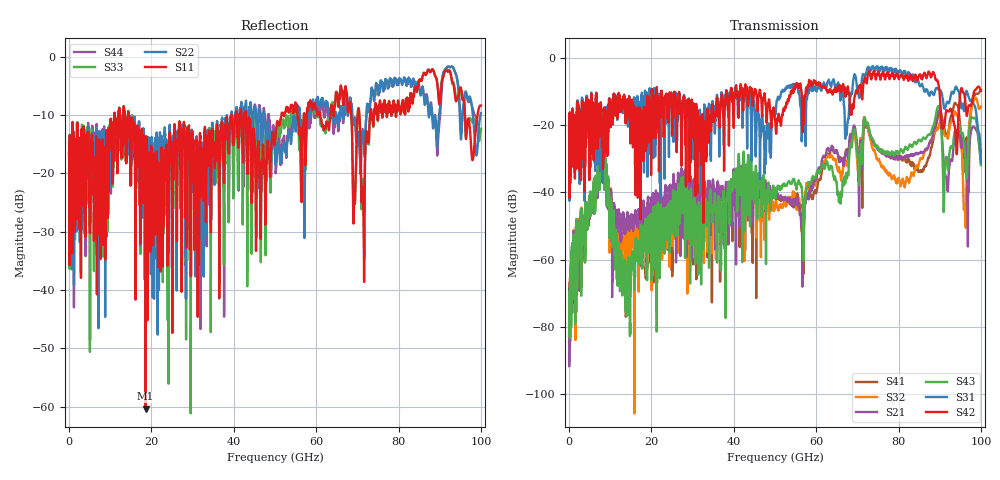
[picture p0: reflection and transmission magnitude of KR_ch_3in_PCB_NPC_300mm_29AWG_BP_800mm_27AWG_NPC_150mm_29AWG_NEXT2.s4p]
# GHz S RI R 45
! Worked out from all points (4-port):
!   4000 points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, 25 MHz to 100 GHz, reference 45 ohm
!   strongest paths, dB at 25 MHz, 25.02 GHz, 50.02 GHz, 75.03 GHz, 100 GHz:
!     S42: -21.2, -20.7, -18.6, -4.1, -9.8
!     S31: -21.2, -17.2, -16.6, -3.0, -31.1
!     S43: -82.6, -50.9, -40.6, -26.3, -31.8
!     S21: -81.4, -46.9, -40.6, -27.2, -27.3
!     S32: -84.4, -52.2, -44.9, -30.5, -14.5
!     S41: -90.0, -64.8, -40.8, -27.2, -9.6
!   lowest |S11| = -60.3 dB at 18.6 GHz (marker M1), VSWR 1.00, Z = 44.9 - j0.04 ohm
!   |S11| at or under -10 dB: start of sweep to 11.02 GHz; 14.45 GHz to 39.38 GHz (24.93 GHz wide, 92.6 % of centre); 42.93 GHz to 51.57 GHz (8.639 GHz wide, 18.3 % of centre)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
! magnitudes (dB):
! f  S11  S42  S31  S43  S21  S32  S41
! 25 MHz  -16.6  -21.2  -21.2  -82.6  -81.4  -84.4  -90.0
! 8.025 GHz  -15.9  -26.5  -21.6  -24.9  -26.1  -25.9  -25.5
! 13.62 GHz  -11.5  -13.1  -12.4  -67.3  -52.3  -61.5  -53.4
! 18.6 GHz  -60.3  -19.1  -14.7  -48.9  -53.9  -47.2  -59.2
! 71.95 GHz  -15.2  -6.4  -5.3  -18.8  -19.3  -18.8  -20.1
! 96.1 GHz  -9.6  -11.7  -13.2  -28.5  -24.6  -44.5  -27.3
! 100 GHz  -8.4  -9.8  -31.1  -31.8  -27.3  -14.5  -9.6
